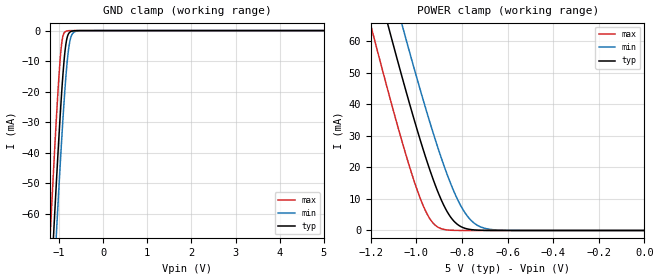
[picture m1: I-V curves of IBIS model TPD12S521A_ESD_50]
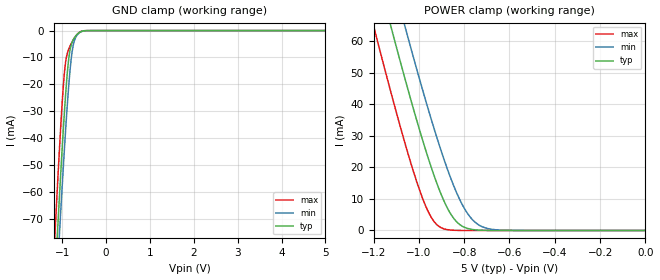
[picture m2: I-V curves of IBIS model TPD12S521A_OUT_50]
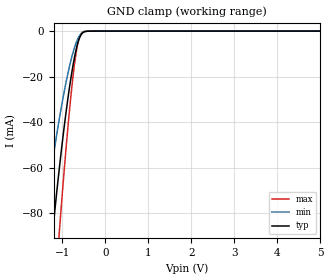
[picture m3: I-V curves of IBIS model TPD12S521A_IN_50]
| TEXAS INSTRUMENTS INCORPORATED
| Standard Linear and Logic Group / High Volume Linear
| IBIS Model of TPD12S521
| SINGLE-CHIP HDMI TRANSMITTER PORT PROTECTION AND INTERFACE DEVICE
| This file contains package information for the following:
|  TSSOP 38-pin (DBT) package as [Component] TPD12S521_DBT
| This device can be powered at the following Vccs:
|  5 volt Vcc
| This file provides unique models under the [Model Selector] for each Vcc.
| For operation at a specific Vcc, select the appropriate model after each
| [Model Selector] keyword.
[IBIS Ver]   3.2
[Comment char]  |_char
[File Name]   tpd12s521.ibs
[File Rev]   1.0 | x_die
[Date]   August 4, 2010
[Source]   Data created from TI-SPICE simulations at TI-SLL/HVL.
   The following is an IBIS list for the TPD12S521.
   Please contact sllibis@ti.com with questions and
   comments concerning SLL IBIS models.
[Notes]   Revision_History:
   Series_MOSFET data is non-monotonic
   TPD12S521A_OUT_50_S: Series MOSFET has decreasing current
[Disclaimer]
| This model is designed as an aid for customers of Texas Instruments.
| TI and its licensors and suppliers make no warranties, either expressed
| or implied, with respect to this  model, including the warranties of
| merchantability or fitness for a particular purpose. The model is
| provided solely on an "as is" basis. The entire risk as to its quality
| and performance is with the customer.
[Copyright]
| (C) Copyright 2010 Texas Instruments Incorporated. All rights reserved.
| Component TPD12S521_DBT 38-PIN TSSOP
[Component]   TPD12S521_DBT
[Manufacturer]   Texas Instruments, Inc.
[Package]
|   typ   min   max
R_pkg   5.900e-02   4.300e-02   8.100e-02
L_pkg   2.296e-09   1.559e-09   3.814e-09
C_pkg   4.140e-13   2.740e-13   7.120e-13
[Pin]   signal_name   model_name   R_pin   L_pin   C_pin
1   VCC   POWER   7.700e-02   3.718e-09   7.100e-13
2   LV_SUPPLY  POWER   7.300e-02   3.331e-09   7.020e-13
3   GND   GND   7.000e-02   2.959e-09   5.760e-13
4   TMDS_D2P   TPD12S521A_ESD_50   6.200e-02   2.225e-09   3.800e-13
5   GND   GND   5.500e-02   1.852e-09   3.070e-13
6   TMDS_D2N   TPD12S521A_ESD_50   5.000e-02   1.734e-09   2.820e-13
7   TMDS_D1P   TPD12S521A_ESD_50   4.700e-02   1.668e-09   2.780e-13
8   GND   GND   4.500e-02   1.612e-09   2.750e-13
9   TMDS_D1N   TPD12S521A_ESD_50   4.300e-02   1.559e-09   2.740e-13
10   TMDS_D0P   TPD12S521A_ESD_50   4.300e-02   1.562e-09   2.750e-13
11   GND   GND   4.400e-02   1.601e-09   2.760e-13
12   TMDS_D0N   TPD12S521A_ESD_50   4.500e-02   1.612e-09   2.760e-13
13   TMDS_CKP   TPD12S521A_ESD_50   4.700e-02   1.668e-09   2.780e-13
14   GND   GND   5.000e-02   1.734e-09   2.820e-13
15   TMDS_CKN   TPD12S521A_ESD_50   5.500e-02   1.852e-09   3.100e-13
16   CE_REMOTE_IN TPD12S521A_IN_50   6.200e-02   2.225e-09   3.820e-13
17   DDC_CLK_IN TPD12S521A_IN_50   7.000e-02   2.958e-09   5.770e-13
18   DDC_DAT_IN TPD12S521A_IN_50   7.300e-02   3.332e-09   7.080e-13
19   HOTPLUG_DET_IN TPD12S521A_IN_50 7.700e-02   3.720e-09   6.970e-13
20   HOTPLUG_DET_OUT TPD12S521A_OUT_50 8.100e-02   3.809e-09   6.940e-13
21   DDC_DAT_OUT TPD12S521A_OUT_50   7.600e-02   3.397e-09   6.990e-13
22   DDC_CLK_OUT TPD12S521A_OUT_50   7.000e-02   2.971e-09   5.730e-13
23   CE_REMOTE_OUT TPD12S521A_OUT_50 6.200e-02   2.233e-09   3.770e-13
24   TMDS_CKN   TPD12S521A_ESD_50   6.000e-02   1.986e-09   3.100e-13
25   GND   GND   5.500e-02   1.857e-09   2.890e-13
26   TMDS_CKP   TPD12S521A_ESD_50   5.100e-02   1.752e-09   2.840e-13
27   TMDS_D0N   TPD12S521A_ESD_50   4.700e-02   1.663e-09   2.800e-13
28   GND   GND   4.500e-02   1.625e-09   2.790e-13
29   TMDS_D0P   TPD12S521A_ESD_50   4.700e-02   1.654e-09   2.820e-13
30   TMDS_D1N   TPD12S521A_ESD_50   4.900e-02   1.702e-09   2.840e-13
31   GND   GND   4.700e-02   1.665e-09   2.810e-13
32   TMDS_D1P   TPD12S521A_ESD_50   5.100e-02   1.755e-09   2.840e-13
33   TMDS_D2N   TPD12S521A_ESD_50   5.500e-02   1.857e-09   2.890e-13
34   GND   GND   6.000e-02   1.986e-09   3.100e-13
35   TMDS_D2P   TPD12S521A_ESD_50   6.200e-02   2.232e-09   3.770e-13
36   GND   GND   7.000e-02   2.971e-09   5.740e-13
37   ESD_BYP   POWER   7.600e-02   3.399e-09   7.010e-13
38   5V_OUT   POWER   8.100e-02   3.814e-09   7.120e-13
[Series Switch Groups]
| Function Group States
On  1 /   | CE_REMOTE_IN->CE_REMOTE_OUT LV_SUPPLY HIGH
   | CE_REMOTE_OUT->CE_REMOTE_IN LV_SUPPLY HIGH
On  2 /   | DDC_CLK_IN->DDC_CLK_OUT LV_SUPPLY HIGH
   | DDC_CLK_OUT->DDC_CLK_IN LV_SUPPLY HIGH
On  3 /   | DDC_DAT_IN->DDC_DAT_OUT LV_SUPPLY HIGH
   | DDC_DAT_OUT->DDC_DAT_IN LV_SUPPLY HIGH
On  4 /   | HOTPLUG_DET_IN->HOTPLUG_DET_OUT LV_SUPPLY HIGH
   | HOTPLUG_DET_OUT->HOTPLUG_DET_IN LV_SUPPLY HIGH
Off 1 2 3 4  /   | LV_SUPPLY LOW
[Series Pin Mapping]   pin_2   model_name   function_table_group
16   23   TPD12S521A_IN_50_S   1
23   16   TPD12S521A_OUT_50_S   1
17   22   TPD12S521A_IN_50_S   2
22   17   TPD12S521A_OUT_50_S   2
18   21   TPD12S521A_IN_50_S   3
21   18   TPD12S521A_OUT_50_S   3
19   20   TPD12S521A_IN_50_S   4
20   19   TPD12S521A_OUT_50_S   4
[Model]   TPD12S521A_OUT_50_S
Model_type  Series_switch
| variable   typ   min   max
C_comp   0   0   0
[Temperature Range]   40   100   -40
| Ambient temperature   25   85   -40
[Voltage range]   5   4.5   5.5
[On]
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[Off]
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[Model]   TPD12S521A_IN_50_S
Model_type  Series_switch
| variable   typ   min   max
C_comp   0   0   0
[Temperature Range]   40   100   -40
| Ambient temperature   25   85   -40
[Voltage range]   5   4.5   5.5
[On]
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[Off]
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| Models and submodels in the file (5): TPD12S521A_ESD_50 (Input), TPD12S521A_OUT_50_S (Series_switch), TPD12S521A_OUT_50 (Terminator), TPD12S521A_IN_50_S (Series_switch), TPD12S521A_IN_50 (Terminator)
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| Model TPD12S521A_ESD
| Model TPD12S521A_OUT
| Model TPD12S521A_OUT_S
| Model TPD12S521A_IN
| Model TPD12S521A_IN_S
[Model]   TPD12S521A_ESD_50
Model_type  Input
Vinl=0.8
Vinh=2.0
| variable   typ   min   max
C_comp   0.65pF   0.60pF   0.77pF
[Temperature Range]   40   100   -40
| Ambient temperature   25   85   -40
[Voltage range]   5   4.5   5.5
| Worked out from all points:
|   GND clamp passes 1 mA (typ) near -0.78 V on its own axis
|   POWER clamp passes 1 mA (typ) near -0.80 V on its own axis
[GND Clamp]
| TPD12S521A_ESD_50
|   Voltage   I(typ)   I(min)   I(max)
-5V       -1.252A    -1.266A    -1.235A
-1.205V   -89.29mA   -106.5mA   -67.88mA
-1.18V    -82.21mA   -99.38mA   -60.8mA
-1.12V    -65.48mA   -82.58mA   -44.16mA
-1.055V   -47.94mA   -64.83mA   -27.09mA
-990mV    -31.4mA    -47.75mA   -12.15mA
-945mV    -20.97mA   -36.54mA   -4.681mA
-845mV    -4.345mA   -14.92mA   -232.8uA
-790mV    -1.15mA    -6.666mA   -44.29uA
-745mV    -407.6uA   -2.797mA   -6.492uA
-605mV    -9.44uA    -173.3uA   -6.672nA
5V        15pA       1.91uA     14.5pA
[POWER Clamp]
| TPD12S521A_ESD_50
|   Voltage   I(typ)   I(min)   I(max)
-5V       1.232A     1.246A     1.215A
-1.21V    88.51mA    105.3mA    67.6mA
-1.19V    82.93mA    99.71mA    62.01mA
-1.13V    66.4mA     83.13mA    45.55mA
-1.11V    60.98mA    77.68mA    40.2mA
-1.065V   49.04mA    65.59mA    28.57mA
-985mV    28.99mA    44.9mA     10.46mA
-930mV    16.81mA    31.61mA    2.587mA
-845mV    3.738mA    13.95mA    67.29uA
-750mV    195uA      2.506mA    745.3nA
-640mV    4.073uA    120.5uA    4.026nA
0V        0A         0A         0A
[Model]   TPD12S521A_OUT_50
Model_type  Terminator
| variable   typ   min   max
C_comp   1.60pF   1.38pF   1.97pF
| C_tri-state   1.60pF   1.38pF   1.97pF
[Temperature Range]   40   100   -40
| Ambient temperature   25   85   -40
[Voltage range]   5   4.5   5.5
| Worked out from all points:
|   GND clamp passes 1 mA (typ) near -0.63 V on its own axis
|   POWER clamp passes 1 mA (typ) near -0.80 V on its own axis
[GND Clamp]
| TPD12S521A_OUT_50
|   Voltage   I(typ)   I(min)   I(max)
-5V       -1.413A    -1.392A    -1.438A
-1.175V   -95.28mA   -108.7mA   -78.42mA
-1.15V    -87.5mA    -101.1mA   -70.4mA
-1.11V    -75.23mA   -89.11mA   -57.82mA
-1.07V    -63.23mA   -77.3mA    -45.66mA
-1.055V   -58.81mA   -72.93mA   -41.25mA
-950mV    -29.97mA   -43.68mA   -15.44mA
-905mV    -19.58mA   -32.24mA   -9.833mA
-845mV    -9.503mA   -18.85mA   -6.583mA
-745mV    -3.267mA   -5.056mA   -3.331mA
-580mV    -451.3uA   -504.2uA   -353.7uA
5V        279.9pA    1.911uA    193.6pA
[POWER Clamp]
| TPD12S521A_OUT_50
|   Voltage   I(typ)   I(min)   I(max)
-5V       1.232A     1.246A     1.215A
-1.21V    88.51mA    105.3mA    67.6mA
-1.19V    82.93mA    99.71mA    62.01mA
-1.13V    66.4mA     83.13mA    45.55mA
-1.11V    60.98mA    77.68mA    40.2mA
-1.065V   49.04mA    65.59mA    28.57mA
-985mV    28.99mA    44.9mA     10.46mA
-930mV    16.81mA    31.61mA    2.587mA
-845mV    3.738mA    13.95mA    67.29uA
-750mV    195uA      2.506mA    745.5nA
-640mV    4.073uA    120.5uA    4.246nA
0V        0A         0A         0A
[Model]   TPD12S521A_IN_50
Model_type  Terminator
| variable   typ   min   max
C_comp   3.51pF   2.96pF   4.18pF
| C_tri-state   3.51pF   2.96pF   4.18pF
[Temperature Range]   40   100   -40
| Ambient temperature   25   85   -40
[Voltage range]   5   4.5   5.5
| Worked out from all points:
|   GND clamp passes 1 mA (typ) near -0.54 V on its own axis
[GND Clamp]
| TPD12S521A_IN_50
|   Voltage   I(typ)   I(min)   I(max)
-5V       -1.074A    -812.4mA   -1.353A
-1.47V    -137.5mA   -90.44mA   -197.5mA
-1.42V    -126.9mA   -83.17mA   -183mA
-1.225V   -87.91mA   -56.78mA   -128.2mA
-1.08V    -61.7mA    -39.43mA   -90.3mA
-1.06V    -58.31mA   -37.2mA    -85.31mA
-895mV    -32.74mA   -20.62mA   -47.1mA
-800mV    -20.34mA   -12.73mA   -28.09mA
-730mV    -12.61mA   -7.908mA   -16.16mA
-625mV    -4.174mA   -2.784mA   -4.066mA
-510mV    -503.3uA   -423.2uA   -254.7uA
5V        519.7pA    1.512nA    166.2pA
